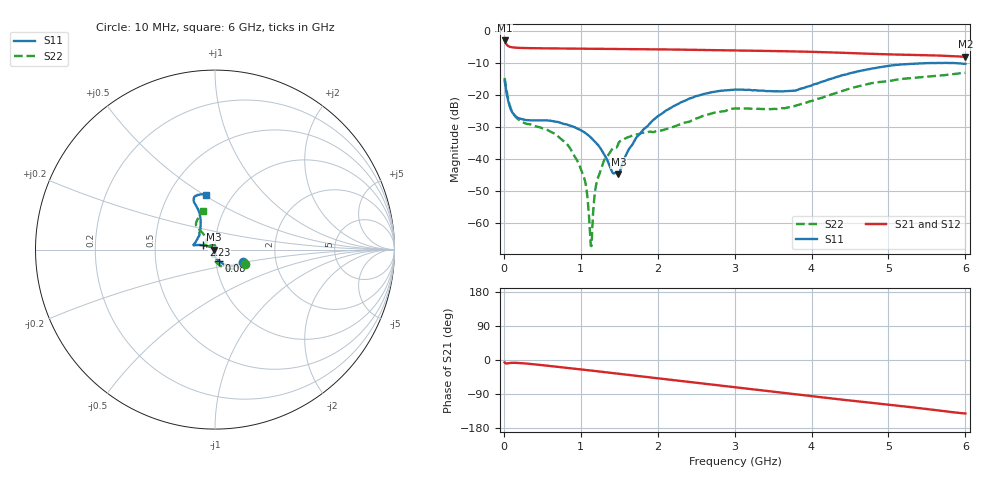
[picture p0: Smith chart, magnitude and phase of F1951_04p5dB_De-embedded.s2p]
! Integrated Device Technology
! Corporate Headquarters
! 6024 Silver Creek Valley Road
! San Jose, CA 95138  USA
! Phone:  1-408-284-8200
! Toll Free:  1-800-223-1366
! Webpage:  http://www.idt.com/
! Timing and RF Division
! 515 Groton Road, Suite 102
! Westford, MA 01886-6024
! Device:  F1951
! Description: 6-bit 0.5 dB Digital Step Attenuator
! Frequency:  100.0 -  4000.00 MHz
! Package:  4x4 mm Thin QFN Plastic Package: 24 pin
! Ports:  2 RF, 6 DC
!  Pin  1  = NC
!  Pin  2  = RF1  =  Port 1
!  Pin  3  = GND
!  Pin  4  = NC
!  Pin  5  = Serial Data Out (SDO)
!  Pin  6  = NC
!  Pin  7  = Reset Bar ( RSTb)
!  Pin  8  = Clock (CLK)
!  Pin  9  = Chip Select Bar (CSb)
!  Pin 10  = NC
!  Pin 11  = Serial Data In (SDI)
!  Pin 12  = NC
!  Pin 13  = NC
!  Pin 14  = VDD
!  Pin 15  = NC
!  Pin 16  = GND
!  Pin 17  = RF2  =  Port 2
!  Pin 18  = NC
!  Pin 19  = GND
!  Pin 20  = GND
!  Pin 21  = GND
!  Pin 22  = GND
!  Pin 23  = GND
!  Pin 24  = GND
! State:  9
! Atten State:  4.5 dB
! Voltage:  +3.30 Volts
! Current:  0.488 mA
! Data:  The device was measured on a F195X evaluation board which has
!  individual transmission lines to the RF pins.  Data was collected
!  de-embedded using a Automatic Fixture Removal [AFR] (Keysight Technologies).
!  The reference plane is the edge of the package pin.
! Misc:  Lot Code  1225BCA
!  Action Tracker AT0399
! Date Measured:  2018-09-13
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# GHz S dB R 50
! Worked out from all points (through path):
!   600 points, 10 MHz to 6 GHz, reference 50 ohm
!   highest |S21| = -2.89 dB at 10 MHz (marker M1); lowest = -8.0 dB at 6 GHz (marker M2)
!   group delay of S21, straight-line fit = 64.3 ps
!   lowest |S11| = -44.8 dB at 1.49 GHz (marker M3), VSWR 1.01, Z = 49.4 - j0.101 ohm
!   |S11| at or under -10 dB: start of sweep to 5.473 GHz; 5.485613 GHz to 5.51034 GHz (24.73 MHz wide, 0.45 % of centre); 5.872 GHz to end of sweep
!   |S22| runs from -67.2 to -13.0 dB; largest |S21 - S12| = 0.00072
!   S11 on the Smith chart (normalised r, x): 10 MHz: 1.35, -0.20; 80 MHz: 1.03, -0.13; 2.23 GHz: 0.88, +0.04; 6 GHz: 0.75, +0.51
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0.01  -15.41 -25.0  -2.89 -6.1  -2.89 -6.1  -14.62 -25.6
0.08  -23.73 -71.6  -4.88 -7.8  -4.88 -7.9  -23.41 -86.9
0.21  -27.34 -88.6  -5.21 -8.1  -5.21 -8.1  -27.88 -110.9
0.8  -29.06 -89.1  -5.40 -20.3  -5.41 -20.3  -34.79 -117.0
1.01  -31.07 -84.0  -5.46 -25.1  -5.46 -25.1  -43.70 -110.7
1.06  -31.81 -84.7  -5.46 -26.3  -5.46 -26.2  -47.29 -108.4
1.11  -32.78 -84.6  -5.47 -27.3  -5.47 -27.3  -58.75 -112.9
1.13  -33.23 -85.0  -5.47 -27.8  -5.47 -27.8  -67.05 -161.3
1.15  -33.70 -85.1  -5.47 -28.3  -5.47 -28.3  -61.49 94.4
1.2  -34.90 -86.7  -5.48 -29.4  -5.48 -29.4  -48.02 79.1
1.25  -36.38 -88.4  -5.48 -30.6  -5.49 -30.6  -44.18 79.4
1.41  -44.11 -118.2  -5.52 -34.4  -5.52 -34.4  -36.83 80.5
1.49  -44.75 -169.8  -5.55 -36.1  -5.55 -36.2  -35.07 89.0
1.72  -33.37 150.8  -5.58 -41.7  -5.58 -41.7  -32.30 93.7
2.01  -26.44 155.3  -5.67 -48.6  -5.67 -48.6  -31.03 114.7
2.23  -23.15 160.0  -5.74 -53.9  -5.74 -53.9  -29.71 135.2
2.59  -19.66 165.9  -5.87 -62.4  -5.87 -62.4  -26.49 158.7
3.01  -18.26 168.6  -6.04 -72.2  -6.04 -72.2  -24.15 163.3
3.65  -18.74 145.6  -6.26 -87.2  -6.26 -87.2  -24.08 139.0
4.01  -16.84 124.4  -6.45 -95.8  -6.45 -95.7  -21.78 127.5
5.01  -10.83 113.9  -7.25 -118.1  -7.25 -118.1  -15.57 127.9
6  -10.21 99.6  -8.00 -141.2  -8.00 -141.2  -13.00 107.4
